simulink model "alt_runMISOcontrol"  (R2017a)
settings: Solver=VariableStepAuto  StartTime=0.0  StopTime=150  RelTol=1e-3
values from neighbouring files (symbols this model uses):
  altu1_threshold = 0.2    [MISOcontrol.m]    (also in init.m = 0)
  altu2_threshold = 0.2    [MISOcontrol.m]    (also in init.m = 0)
  baud = 250000    [MISOcontrol.m]    (also in MISO_demo.m; runSteptest.m; SISOcontrol.m; init.m)
  bo_c21 = +0.1    (= 0.1)    [MISOcontrol.m]    (also in MISO_demo.m = 0.15; MIMOcontrol.m)
  com = 'COM4'    [MISOcontrol.m]    (also in MISO_demo.m; runSteptest.m; SISOcontrol.m; init.m)
  fixed_u1 = 0    [MISOcontrol.m]    (also in MISO_demo.m; SISOcontrol.m; init.m)
  fixed_u2 = 0    [MISOcontrol.m]    (also in MISO_demo.m; SISOcontrol.m; init.m)
  fixed_u3 = 0    [MISOcontrol.m]    (also in MISO_demo.m; SISOcontrol.m; init.m)
  fTf = 0.1    [MISOcontrol.m]    (also in MISO_demo.m; runSteptest.m; SISOcontrol.m; init.m)
  fTl = 0.05    [MISOcontrol.m]    (also in MISO_demo.m; runSteptest.m; SISOcontrol.m; init.m)
  fTt = 0.05    [MISOcontrol.m]    (also in MISO_demo.m; runSteptest.m; SISOcontrol.m; init.m)
  step_d1 = -2.5    [MISOcontrol.m]    (also in MISO_demo.m; SISOcontrol.m = -2; init.m = 0)
  step_d2 = +2.5    (= 2.5)    [MISOcontrol.m]    (also in MISO_demo.m; SISOcontrol.m = 2; init.m = 0)
  step_ys1 = 5    [MISOcontrol.m]    (also in MISO_demo.m; SISOcontrol.m = 4)
  step_ys2 = -5    [MISOcontrol.m]    (also in MISO_demo.m; SISOcontrol.m = -4)
  stepTime_d1 = 90    [MISOcontrol.m]    (also in MISO_demo.m; SISOcontrol.m = 6; init.m = 0)
  stepTime_d2 = 120    [MISOcontrol.m]    (also in MISO_demo.m; SISOcontrol.m = 8; init.m = 0)
  stepTime_ys1 = 30    [MISOcontrol.m]
  stepTime_ys2 = 60    [MISOcontrol.m]
  Ts = 0.1    [identification.m]    (also in MISOcontrol.m; MISO_demo.m; runSteptest.m; SISOcontrol.m)
  turnOn_y1 = 1    [MISOcontrol.m]    (also in MISO_demo.m; SISOcontrol.m = 0)
  turnOn_y2 = 0    [MISOcontrol.m]    (also in MISO_demo.m; SISOcontrol.m = 1)
  y0 = sb_T+3    (= 30)    [MISOcontrol.m]    (also in MISO_demo.m = sb_T; SISOcontrol.m = 0; init.m = 0; MIMOcontrol.m = 27)
  y_s0 = 0    [MISOcontrol.m]    (also in MISO_demo.m; SISOcontrol.m = 4)
undefined symbols (not defined in the file or in its folder): alt_Kc11, alt_Kc21, alt_tauI11, alt_tauI21, Kb, Kc11, Kc21, tauI11, tauI21
libraries: simulink x4, tom_lib x1

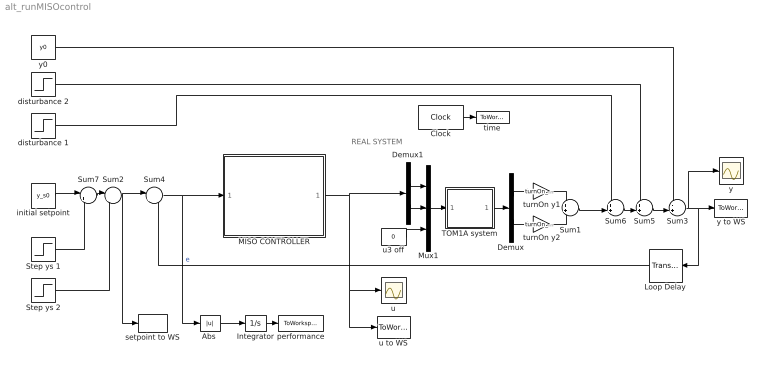
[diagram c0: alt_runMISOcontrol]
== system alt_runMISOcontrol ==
  note: REAL SYSTEM
  "Abs " : Abs  ZeroCross=off
  Clock : Clock
  Demux : Demux  Outputs=2
  Demux1 : Demux  Outputs=2
  Integrator : Integrator  ZeroCross=off
  Loop Delay : TransportDelay  DelayTime=0.1
  MISO CONTROLLER : Subsystem
  Mux1 : Mux  Inputs=3
  Step ys 1 : Step  Time=stepTime_ys1  After=step_ys1  SampleTime=Ts  ZeroCross=off
  Step ys 2 : Step  Time=stepTime_ys2  After=step_ys2  SampleTime=Ts  ZeroCross=off
  Sum1 : Sum
  Sum2 : Sum  Inputs=|++
  Sum3 : Sum  Inputs=-+|
  Sum4 : Sum  Inputs=|+-
  Sum5 : Sum  Inputs=++|
  Sum6 : Sum  Inputs=++|
  Sum7 : Sum  Inputs=|++
  TOM1A system : Subsystem
  disturbance 1 : Step  Time=stepTime_d1  After=step_d1  SampleTime=Ts  ZeroCross=off
  disturbance 2 : Step  Time=stepTime_d2  After=step_d2  SampleTime=Ts  ZeroCross=off
  initial setpoint : Constant  Value=y_s0  SampleTime=Ts
  performance : ToWorkspace  VariableName=IAE  SampleTime=Ts
  setpoint to WS : ToWorkspace  VariableName=ys  SampleTime=Ts
  time : ToWorkspace  VariableName=time  SampleTime=Ts
  turnOn y1 : Gain  Gain=turnOn_y1
  turnOn y2 : Gain  Gain=turnOn_y2
  u : Scope
  u to WS : ToWorkspace  VariableName=u  SampleTime=Ts
  u3 off : Constant  Value=0  SampleTime=Ts
  y : Scope
  y to WS : ToWorkspace  VariableName=y  SampleTime=Ts
  y0 : Constant  Value=y0  SampleTime=Ts
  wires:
  Clock/1 -> time/1
  disturbance 1/1 -> Sum6/1
  Sum3/1 -> y/1, Loop Delay/1, y to WS/1
  "Abs "/1 -> Integrator/1
  TOM1A system/1(y) -> Demux/1
  Integrator/1 -> performance/1
  Mux1/1 -> TOM1A system/1(u)
  u3 off/1 -> Mux1/3
  Demux/1 -> turnOn y1/1
  Demux/2 -> turnOn y2/1
  turnOn y2/1 -> Sum1/2
  turnOn y1/1 -> Sum1/1
  Loop Delay/1 -> Sum4/2
  Sum1/1 -> Sum6/2
  Sum6/1 -> Sum5/2
  disturbance 2/1 -> Sum5/1
  Sum5/1 -> Sum3/2
  y0/1 -> Sum3/1
  initial setpoint/1 -> Sum7/1
  Step ys 2/1 -> Sum2/2
  Sum7/1 -> Sum2/1
  Step ys 1/1 -> Sum7/2
  Sum2/1 -> Sum4/1, setpoint to WS/1
  Sum4/1 -> "Abs "/1, MISO CONTROLLER/1(e)  "e"
  Demux1/1 -> Mux1/1
  Demux1/2 -> Mux1/2
  MISO CONTROLLER/1(u) -> u to WS/1, u/1, Demux1/1

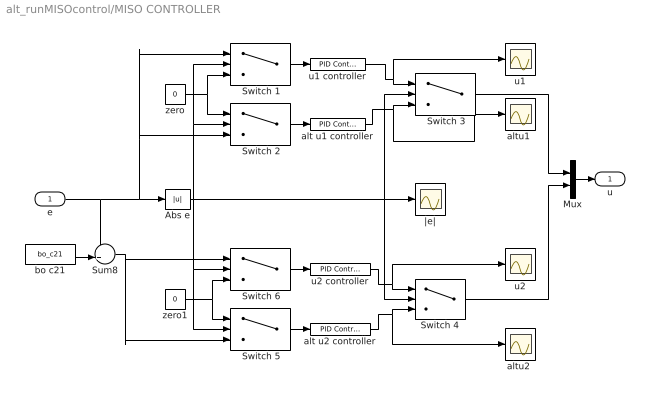
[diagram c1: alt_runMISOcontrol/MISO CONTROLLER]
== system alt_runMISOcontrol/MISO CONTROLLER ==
  e : Inport
  " Switch 1" : Switch  Criteria=u2 > Threshold  Threshold=altu1_threshold  ZeroCross=off
  " Switch 2" : Switch  Criteria=u2 > Threshold  Threshold=altu1_threshold  ZeroCross=off
  " Switch 3" : Switch  Criteria=u2 > Threshold  Threshold=altu1_threshold  ZeroCross=off
  " Switch 5" : Switch  Criteria=u2 > Threshold  Threshold=altu2_threshold  ZeroCross=off
  " Switch 6" : Switch  Criteria=u2 > Threshold  Threshold=altu2_threshold  ZeroCross=off
  Abs e : Abs  ZeroCross=off
  Mux : Mux  Inputs=2
  Sum8 : Sum  Inputs=++|
  Switch 4 : Switch  Criteria=u2 > Threshold  Threshold=altu2_threshold  ZeroCross=off
  alt u1 controller : simulink/Continuous/PID Controller  Controller=PI  TimeDomain=Discrete-time  SampleTime=Ts  IntegratorMethod=Forward Euler  FilterMethod=Forward Euler  Form=Parallel  UseFilter=on  ControllerParametersSource=internal  P=alt_Kc11  I=alt_Kc11/alt_tauI11  D=0  N=100  InitialConditionSource=internal  InitialConditionForIntegrator=0  InitialConditionForFilter=0  ExternalReset=none  ZeroCross=off  LimitOutput=on  UpperSaturationLimit=1  LowerSaturationLimit=0  LinearizeAsGain=on  AntiWindupMode=clamping  Kb=Kb  TrackingMode=off  Kt=1  PParamMin=[]  PParamMax=[]  IParamMin=[]  IParamMax=[]  DParamMin=[]  DParamMax=[]  NParamMin=[]  NParamMax=[]  KbParamMin=[]  KbParamMax=[]  KtParamMin=[]  KtParamMax=[]  POutMin=[]  POutMax=[]  IOutMin=[]  IOutMax=[]  DOutMin=[]  DOutMax=[]  NOutMin=[]  NOutMax=[]  KbOutMin=[]  KbOutMax=[]  KtOutMin=[]  KtOutMax=[]  IntegratorOutMin=[]  IntegratorOutMax=[]  FilterOutMin=[]  FilterOutMax=[]  SumOutMin=[]  SumOutMax=[]  SumI1OutMin=[]  SumI1OutMax=[]  SumI2OutMin=[]  SumI2OutMax=[]  SumI3OutMin=[]  SumI3OutMax=[]  SumDOutMin=[]  SumDOutMax=[]  SaturationOutMin=[]  SaturationOutMax=[]  IntegratorContinuousStateAttributes=''  IntegratorStateMustResolveToSignalObject=off  IntegratorRTWStateStorageClass=Auto  FilterContinuousStateAttributes=''  FilterStateMustResolveToSignalObject=off  FilterRTWStateStorageClass=Auto  DifferentiatorICPrevScaledInput=0  DifferentiatorOutMin=[]  DifferentiatorOutMax=[]  InitialConditionSetting=State (most efficient)
  alt u2 controller : simulink/Continuous/PID Controller  Controller=PI  TimeDomain=Discrete-time  SampleTime=Ts  IntegratorMethod=Forward Euler  FilterMethod=Forward Euler  Form=Parallel  UseFilter=on  ControllerParametersSource=internal  P=alt_Kc21  I=alt_Kc21/alt_tauI21  D=0  N=100  InitialConditionSource=internal  InitialConditionForIntegrator=0  InitialConditionForFilter=0  ExternalReset=none  ZeroCross=off  LimitOutput=on  UpperSaturationLimit=1  LowerSaturationLimit=0  LinearizeAsGain=on  AntiWindupMode=clamping  Kb=Kb  TrackingMode=off  Kt=1  PParamMin=[]  PParamMax=[]  IParamMin=[]  IParamMax=[]  DParamMin=[]  DParamMax=[]  NParamMin=[]  NParamMax=[]  KbParamMin=[]  KbParamMax=[]  KtParamMin=[]  KtParamMax=[]  POutMin=[]  POutMax=[]  IOutMin=[]  IOutMax=[]  DOutMin=[]  DOutMax=[]  NOutMin=[]  NOutMax=[]  KbOutMin=[]  KbOutMax=[]  KtOutMin=[]  KtOutMax=[]  IntegratorOutMin=[]  IntegratorOutMax=[]  FilterOutMin=[]  FilterOutMax=[]  SumOutMin=[]  SumOutMax=[]  SumI1OutMin=[]  SumI1OutMax=[]  SumI2OutMin=[]  SumI2OutMax=[]  SumI3OutMin=[]  SumI3OutMax=[]  SumDOutMin=[]  SumDOutMax=[]  SaturationOutMin=[]  SaturationOutMax=[]  IntegratorContinuousStateAttributes=''  IntegratorStateMustResolveToSignalObject=off  IntegratorRTWStateStorageClass=Auto  FilterContinuousStateAttributes=''  FilterStateMustResolveToSignalObject=off  FilterRTWStateStorageClass=Auto  DifferentiatorICPrevScaledInput=0  DifferentiatorOutMin=[]  DifferentiatorOutMax=[]  InitialConditionSetting=State (most efficient)
  "altu1 " : Scope
  "altu2 " : Scope
  bo c21 : Constant  Value=bo_c21  SampleTime=Ts
  u1 : Scope
  u1 controller : simulink/Continuous/PID Controller  Controller=PI  TimeDomain=Discrete-time  SampleTime=Ts  IntegratorMethod=Forward Euler  FilterMethod=Forward Euler  Form=Parallel  UseFilter=on  ControllerParametersSource=internal  P=Kc11  I=Kc11/tauI11  D=0  N=100  InitialConditionSource=internal  InitialConditionForIntegrator=0  InitialConditionForFilter=0  ExternalReset=none  ZeroCross=off  LimitOutput=on  UpperSaturationLimit=1  LowerSaturationLimit=0  LinearizeAsGain=on  AntiWindupMode=clamping  Kb=Kb  TrackingMode=off  Kt=1  PParamMin=[]  PParamMax=[]  IParamMin=[]  IParamMax=[]  DParamMin=[]  DParamMax=[]  NParamMin=[]  NParamMax=[]  KbParamMin=[]  KbParamMax=[]  KtParamMin=[]  KtParamMax=[]  POutMin=[]  POutMax=[]  IOutMin=[]  IOutMax=[]  DOutMin=[]  DOutMax=[]  NOutMin=[]  NOutMax=[]  KbOutMin=[]  KbOutMax=[]  KtOutMin=[]  KtOutMax=[]  IntegratorOutMin=[]  IntegratorOutMax=[]  FilterOutMin=[]  FilterOutMax=[]  SumOutMin=[]  SumOutMax=[]  SumI1OutMin=[]  SumI1OutMax=[]  SumI2OutMin=[]  SumI2OutMax=[]  SumI3OutMin=[]  SumI3OutMax=[]  SumDOutMin=[]  SumDOutMax=[]  SaturationOutMin=[]  SaturationOutMax=[]  IntegratorContinuousStateAttributes=''  IntegratorStateMustResolveToSignalObject=off  IntegratorRTWStateStorageClass=Auto  FilterContinuousStateAttributes=''  FilterStateMustResolveToSignalObject=off  FilterRTWStateStorageClass=Auto  DifferentiatorICPrevScaledInput=0  DifferentiatorOutMin=[]  DifferentiatorOutMax=[]  InitialConditionSetting=State (most efficient)
  u2 : Scope
  u2 controller : simulink/Continuous/PID Controller  Controller=PI  TimeDomain=Discrete-time  SampleTime=Ts  IntegratorMethod=Forward Euler  FilterMethod=Forward Euler  Form=Parallel  UseFilter=on  ControllerParametersSource=internal  P=Kc21  I=Kc21/tauI21  D=0  N=100  InitialConditionSource=internal  InitialConditionForIntegrator=0  InitialConditionForFilter=0  ExternalReset=none  ZeroCross=off  LimitOutput=on  UpperSaturationLimit=1  LowerSaturationLimit=0  LinearizeAsGain=on  AntiWindupMode=clamping  Kb=Kb  TrackingMode=off  Kt=1  PParamMin=[]  PParamMax=[]  IParamMin=[]  IParamMax=[]  DParamMin=[]  DParamMax=[]  NParamMin=[]  NParamMax=[]  KbParamMin=[]  KbParamMax=[]  KtParamMin=[]  KtParamMax=[]  POutMin=[]  POutMax=[]  IOutMin=[]  IOutMax=[]  DOutMin=[]  DOutMax=[]  NOutMin=[]  NOutMax=[]  KbOutMin=[]  KbOutMax=[]  KtOutMin=[]  KtOutMax=[]  IntegratorOutMin=[]  IntegratorOutMax=[]  FilterOutMin=[]  FilterOutMax=[]  SumOutMin=[]  SumOutMax=[]  SumI1OutMin=[]  SumI1OutMax=[]  SumI2OutMin=[]  SumI2OutMax=[]  SumI3OutMin=[]  SumI3OutMax=[]  SumDOutMin=[]  SumDOutMax=[]  SaturationOutMin=[]  SaturationOutMax=[]  IntegratorContinuousStateAttributes=''  IntegratorStateMustResolveToSignalObject=off  IntegratorRTWStateStorageClass=Auto  FilterContinuousStateAttributes=''  FilterStateMustResolveToSignalObject=off  FilterRTWStateStorageClass=Auto  DifferentiatorICPrevScaledInput=0  DifferentiatorOutMin=[]  DifferentiatorOutMax=[]  InitialConditionSetting=State (most efficient)
  zero : Constant  Value=0  SampleTime=Ts
  zero1 : Constant  Value=0  SampleTime=Ts
  |e| : Scope
  u : Outport
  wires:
  e/1 -> " Switch 2"/3, " Switch 1"/1, Abs e/1, Sum8/1
  Mux/1 -> u/1
  Abs e/1 -> Switch 4/2, " Switch 3"/2, |e|/1, " Switch 1"/2, " Switch 2"/2, " Switch 5"/2, " Switch 6"/2
  bo c21/1 -> Sum8/2
  alt u2 controller/1 -> "altu2 "/1, Switch 4/3
  u2 controller/1 -> u2/1, Switch 4/1
  Switch 4/1 -> Mux/2
  " Switch 2"/1 -> alt u1 controller/1
  " Switch 1"/1 -> u1 controller/1
  zero/1 -> " Switch 2"/1, " Switch 1"/3
  alt u1 controller/1 -> "altu1 "/1, " Switch 3"/3
  u1 controller/1 -> u1/1, " Switch 3"/1
  " Switch 3"/1 -> Mux/1
  Sum8/1 -> " Switch 5"/3, " Switch 6"/1
  " Switch 5"/1 -> alt u2 controller/1
  " Switch 6"/1 -> u2 controller/1
  zero1/1 -> " Switch 5"/1, " Switch 6"/3

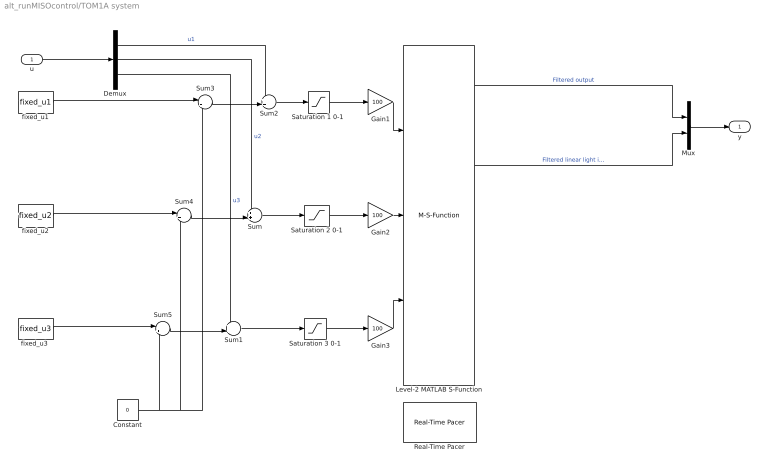
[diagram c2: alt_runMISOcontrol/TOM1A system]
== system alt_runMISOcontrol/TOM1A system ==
  u : Inport
  Constant : Constant  Value=0
  Demux : Demux  Outputs=3
  Gain1 : Gain  Gain=100
  Gain2 : Gain  Gain=100
  Gain3 : Gain  Gain=100
  Level-2 MATLAB S-Function : M-S-Function  FunctionName=tom1ar8  Parameters=Ts,com,baud,fTt,fTl,fTf
  Mux : Mux  Inputs=2
  Real-Time Pacer : tom_lib/Real-Time Pacer  simTimePerRealTime=1
  "Saturation 1 0-1 " : Saturate  UpperLimit=1  LowerLimit=0  ZeroCross=off
  Saturation 2 0-1 : Saturate  UpperLimit=1  LowerLimit=0  ZeroCross=off
  Saturation 3 0-1 : Saturate  UpperLimit=1  LowerLimit=0  ZeroCross=off
  Sum : Sum  Inputs=++|
  Sum1 : Sum  Inputs=++|
  Sum2 : Sum  Inputs=++|
  Sum3 : Sum  Inputs=|++
  Sum4 : Sum  Inputs=|++
  Sum5 : Sum  Inputs=|++
  fixed_u1 : Constant  Value=fixed_u1  SampleTime=Ts
  fixed_u2 : Constant  Value=fixed_u2  SampleTime=Ts
  "fixed_u3 " : Constant  Value=fixed_u3  SampleTime=Ts
  y : Outport
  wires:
  Level-2 MATLAB S-Function/14 -> ?  "Fan filtered  rpm"
  Level-2 MATLAB S-Function/3 -> ?  "Derivative of internal temperature"
  Level-2 MATLAB S-Function/4 -> ?  "Filtered external temperature"
  Level-2 MATLAB S-Function/13 -> ?  "Fan voltage"
  Level-2 MATLAB S-Function/11 -> ?  "Bulb voltage"
  Level-2 MATLAB S-Function/8 -> ?  "Filtered logaritmic light intensity"
  Level-2 MATLAB S-Function/1 -> ?  "Board temperature"
  Level-2 MATLAB S-Function/5 -> ?  "Derivate of external temperature"
  Level-2 MATLAB S-Function/12 -> ?  "Fan current"
  Level-2 MATLAB S-Function/9 -> ?  "Derivate of logaritmic light intensity"
  Level-2 MATLAB S-Function/16 -> ?  "Count of fan rpm"
  Level-2 MATLAB S-Function/15 -> ?  "Derivate of fan rpm"
  Level-2 MATLAB S-Function/10 -> ?  "Bulb current"
  Level-2 MATLAB S-Function/6 -> Mux/2  "Filtered linear light intensity"
  Level-2 MATLAB S-Function/7 -> ?  "Derivate of linear light intensity"
  Demux/1 -> Sum2/1  "u1"
  Demux/2 -> Sum/1  "u2"
  Demux/3 -> Sum1/1  "u3"
  u/1 -> Demux/1
  Level-2 MATLAB S-Function/2 -> Mux/1  "Filtered output"
  Mux/1 -> y/1
  fixed_u1/1 -> Sum3/1
  Sum3/1 -> Sum2/2
  Constant/1 -> Sum5/2, Sum4/2, Sum3/2
  fixed_u2/1 -> Sum4/1
  "fixed_u3 "/1 -> Sum5/1
  Sum5/1 -> Sum1/2
  Sum4/1 -> Sum/2
  Gain1/1 -> Level-2 MATLAB S-Function/1
  Gain2/1 -> Level-2 MATLAB S-Function/2
  Gain3/1 -> Level-2 MATLAB S-Function/3
  Saturation 2 0-1/1 -> Gain2/1
  Sum/1 -> Saturation 2 0-1/1
  "Saturation 1 0-1 "/1 -> Gain1/1
  Sum2/1 -> "Saturation 1 0-1 "/1
  Saturation 3 0-1/1 -> Gain3/1
  Sum1/1 -> Saturation 3 0-1/1
